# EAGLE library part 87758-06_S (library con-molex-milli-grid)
HEADER
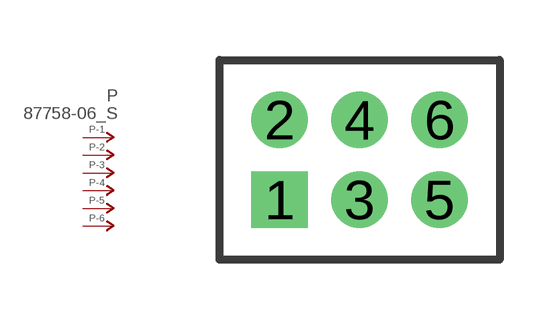
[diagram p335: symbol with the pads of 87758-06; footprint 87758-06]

Designator prefix P; gates -1=P-NV -2=P-N -3=P-N -4=P-N -5=P-N -6=P-N

## 87758-06_S  [87758-06]
1  -1:P  pas
2  -2:P  pas
3  -3:P  pas
4  -4:P  pas
5  -5:P  pas
6  -6:P  pas

## Footprint 87758-06 (pad centres in mm)
HEADER Dual Row, Vertical
drill 0.914 square: 1 -2,-1
drill 0.914: 2 -2,1; 3 0,-1; 4 0,1; 5 2,-1; 6 2,1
